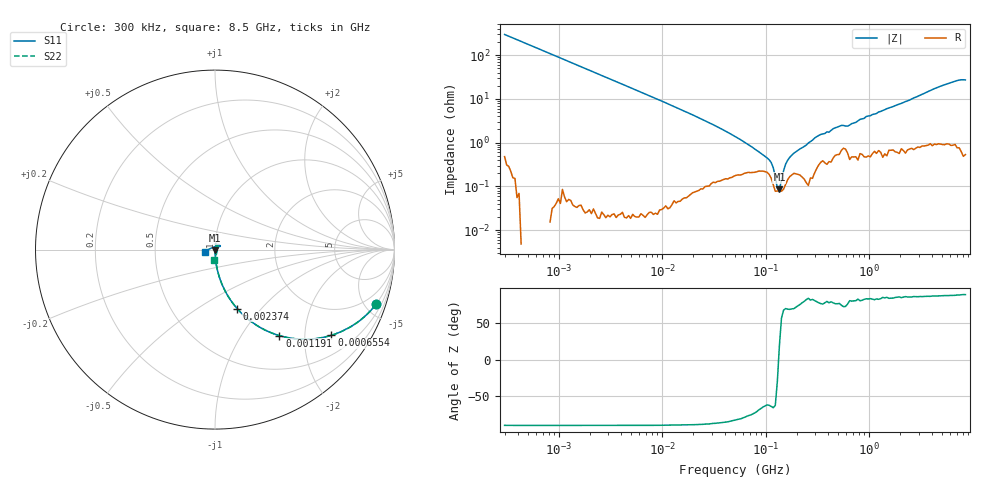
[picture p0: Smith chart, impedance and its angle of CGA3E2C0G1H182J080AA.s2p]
! S-parameter Generated by TDK Corporation
! Copyright(C) 2015 TDK Corporation.
! All Rights Reserved.
! TDK P/N: CGA3E2C0G1H182J080AA (Multilayer Ceramic Chip Capacitors)
! Property: C=1.8nF
! Size(LxWxT): 1.6x0.8x0.8mm, 0.063x0.031x0.031inches
! Model Type: s2p (Touchstone File Format Version 1.0)
! Frequency: DC=Yes Start=0.3MHz Stop=8500MHz 225points Log-sweep
! Note:
! Model Generated on Jun. 23, 2015
! Hash(MD5):
! Port Assignments:
!  1 ---| |--- 2
! Applicable Conditions:
!  Temperature = 25 degC
!  DC Bias Voltage = 0 V
!  Small Signal Operation
! Terms and conditions regarding TDK Simulation Models
! (1)This simulation model is being provided solely for informational purposes. Please refer to the specifications of the products in terms of detailed characteristics of such products.
! (2)In no event shall TDK Corporation of any of its subsidiaries be liable for any loss or damage arising, directly or indirectly,
!  From any information contained in this simulation model, including, but not limited to loss or damages arising from any inaccuracies, omissions or errors in connection with such information.
! (3)Any and all copyrights on this simulation model are owned by TDK Corporation.
!  Duplication or redistribution of this simulation model without prior written permission from TDK Corporation is prohibited.
! (4)This simulation model is subject to any modification or change without any prior notice.
! (5)Neither TDK Corporation nor any of its subsidiaries shall make any warranty, express or implied,
!  Including but not limited to the correctness, implied warranties of merchantability and fitness for a particular purpose with respect to this simulation models.
! (6)The use of this simulation model shall be deemed to have consented to the terms and conditions hereof.
# MHz S MA R 50
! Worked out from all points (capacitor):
!   224 points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, 300 kHz to 8.5 GHz, reference 50 ohm
!   read as one part in series: C = 1.79 nF near 314.1 kHz
!   lowest |Z| = 86 mohm at 135.7 MHz (marker M1)
!   series resonance near 133.3 MHz, so ESL is about 800 pH
!   S11 on the Smith chart (normalised r, x): 300 kHz: 0.99, -5.90; 655.4 kHz: 1.00, -2.71; 1.191 MHz: 1.00, -1.50; 2.374 MHz: 1.00, -0.75; 8.5 GHz: 0.89, -0.02
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0.3  0.9473 -18.7  0.3202 71.2  0.3202 71.3  0.9473 -18.8
0.6554417  0.8051 -36.4  0.5922 53.7  0.5925 53.7  0.8047 -36.4
1.191475  0.5989 -53.2  0.8006 36.8  0.8007 36.8  0.5988 -53.2
1.72111  0.4599 -62.6  0.8878 27.4  0.8879 27.4  0.4598 -62.6
2.374472  0.3515 -69.4  0.936 20.6  0.9361 20.6  0.3514 -69.4
9.430415  0.09328 -84.6  0.9953 5.3  0.9955 5.3  0.09326 -84.4
51.67171  0.01459 -90.5  0.9974 0.6  0.9976 0.6  0.01674 -80.2
135.6836  0.004938 -97.1  0.9977 -0.3  0.9977 -0.3  0.005138 -99.2
283.1228  0.001582 -156.6  0.9952 -1.3  0.995 -1.3  0.002857 138.6
310.3886  0.0005093 128.5  0.9946 -1.4  0.9946 -1.4  0.003499 93.5
356.2888  0.002486 59.9  0.9935 -1.6  0.9935 -1.6  0.003241 67.6
564.2308  0.005573 34.2  0.9899 -2.5  0.9898 -2.4  0.007147 44.0
647.669  0.002517 64.9  0.9924 -2.7  0.9921 -2.8  0.0006611 95.8
710.042  0.0007795 47.9  0.9923 -3.0  0.9921 -3.0  0.005553 57.5
815.0429  0.006496 61.1  0.9923 -3.5  0.9913 -3.6  0.005064 47.9
1025.67  0.003757 78.9  0.9906 -4.5  0.9916 -4.5  0.002499 68.7
1073.923  0.004158 58.3  0.9899 -4.6  0.9907 -4.7  0.00702 77.9
1551.304  0.00625 41.8  0.9899 -6.8  0.9893 -6.6  0.008533 68.0
2456.696  0.004578 82.8  0.9889 -10.5  0.9886 -10.3  0.01015 34.9
4895.91  0.03591 52.6  0.9847 -20.8  0.9837 -20.7  0.03422 71.7
7753.325  0.01614 120.9  0.9841 -33.0  0.9836 -32.7  0.01462 -31.6
8500  0.0573 -167.3  0.9822 -36.0  0.982 -36.0  0.0597 -93.0
